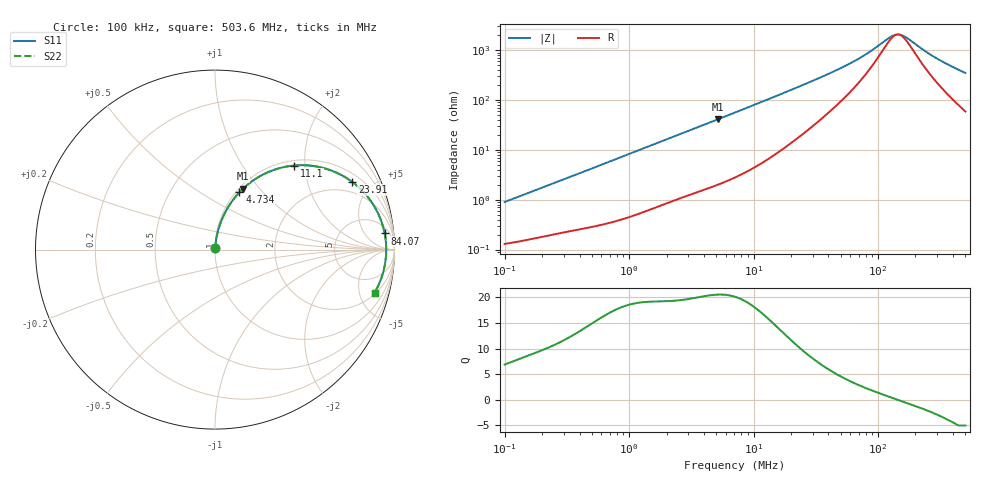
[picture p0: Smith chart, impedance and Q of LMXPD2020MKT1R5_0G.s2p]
! LMXPD2020MKT1R5_0G  S-PARAMETER MODEL  ( General Type )
! Model Generated by TAIYO YUDEN Corporation (http://www.ty-top.com)
! Version 1.0
! TAIYO YUDEN Control No. 191023NI43SB-FBB
! Copyright(c) 2019 TAIYO YUDEN CO.,LTD. All Rights Reserved.
! Product Description (link to TY-COMPAS)
! https://ds.yuden.co.jp/TYCOMPAS/or/detail?pn=LMXPD2020MKT1R5N0G&u=M
! Products Name : Inductors
! Characteristics :
!  Inductance : 1.5 uH , SRF(min) : -Hz , DC Resistance(max) : 0.12 Ohm
!  Rated Current : Saturation :1800 mA , Temp Rise : 1400 mA
!  Case Size : 2.0 x 2.0 / 0.079 x 0.079 [mm/inch] , Thickness : 1.2 / 0.047 [mm/inch]
!  (Conditions: Temperature = 25 degC , DC Bias Current/Voltage = 0A / 0V)
! External Node Assignments :
!  1  o---GGG---o  2
! GND o---------o GND
! Frequency Range : 0.1MHz  -  503.601575MHz  [ 402 STEP ]
# MHz S RI R 50
! Freq[MHz].  S11 Real  S11 Imag  S21 Real  S21 Imag  S12 Real  S12 Imag  S22 Real  S22 Imag
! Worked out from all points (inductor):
!   401 points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, 100 kHz to 503.6 MHz, reference 50 ohm
!   read as one part in series: L = 1.41 uH near 104.4 kHz
!   highest Q = 20.5 at 5.155 MHz (marker M1), where L = 1.26 uH
!   self-resonance near 144.5 MHz
!   S11 on the Smith chart (normalised r, x): 100 kHz: 1.00, +0.02; 4.734 MHz: 1.04, +0.75; 11.1 MHz: 1.10, +1.76; 23.91 MHz: 1.38, +3.83; 84.07 MHz: 9, +16; 503.6 MHz: 2.18, -6.90
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0.1  0.00138 0.00889  0.9986 -0.00889  0.9986 -0.00889  0.00138 0.00889
0.416965  0.00382 0.0351  0.9962 -0.0351  0.9962 -0.0351  0.00382 0.0351
0.917366  0.00986 0.0752  0.9901 -0.0752  0.9901 -0.0752  0.00986 0.0752
1.738598  0.0267 0.1374  0.9733 -0.1374  0.9733 -0.1374  0.0267 0.1374
3.025762  0.0662 0.2244  0.9338 -0.2244  0.9338 -0.2244  0.0662 0.2244
4.733631  0.1362 0.3194  0.8638 -0.3194  0.8638 -0.3194  0.1362 0.3194
5.154841  0.1557 0.339  0.8443 -0.339  0.8443 -0.339  0.1557 0.339
7.249345  0.2584 0.4135  0.7416 -0.4135  0.7416 -0.4135  0.2584 0.4135
11.10205  0.4393 0.4683  0.5607 -0.4683  0.5607 -0.4683  0.4393 0.4683
15.94931  0.6088 0.4533  0.3912 -0.4533  0.3912 -0.4533  0.6088 0.4533
23.91063  0.7656 0.3764  0.2344 -0.3764  0.2344 -0.3764  0.7656 0.3764
29.58987  0.8251 0.3234  0.1749 -0.3234  0.1749 -0.3234  0.8251 0.3234
39.03561  0.8799 0.2532  0.1201 -0.2532  0.1201 -0.2532  0.8799 0.2532
53.73896  0.9187 0.1787  0.0813 -0.1787  0.0813 -0.1787  0.9187 0.1787
84.0715  0.9452 0.0902  0.0548 -0.0902  0.0548 -0.0902  0.9452 0.0902
123.3794  0.9533 0.0254  0.0467 -0.0254  0.0467 -0.0254  0.9533 0.0254
140.2084  0.954 0.00481  0.046 -0.00481  0.046 -0.00481  0.954 0.00481
149.4651  0.954 -0.00543  0.046 0.00543  0.046 0.00543  0.954 -0.00543
159.3329  0.9538 -0.0157  0.0462 0.0157  0.0462 0.0157  0.9538 -0.0157
289.3686  0.9391 -0.1186  0.0609 0.1186  0.0609 0.1186  0.9391 -0.1186
389.964  0.9189 -0.1797  0.0811 0.1797  0.0811 0.1797  0.9189 -0.1797
503.6016  0.8898 -0.2391  0.1102 0.2391  0.1102 0.2391  0.8898 -0.2391
